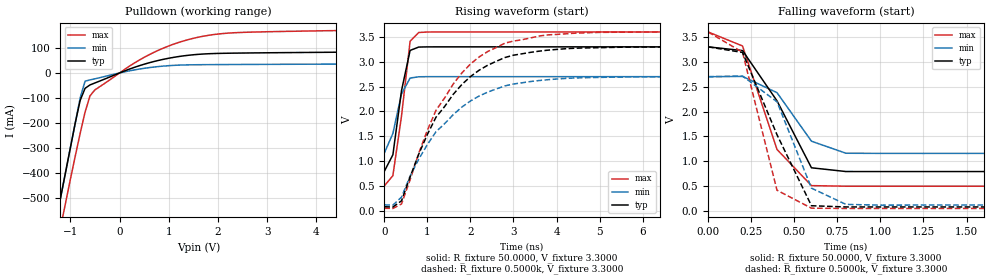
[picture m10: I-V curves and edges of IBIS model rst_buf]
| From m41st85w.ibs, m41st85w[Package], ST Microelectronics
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|   Model rst_buf
[Model]   rst_buf
Model_type   Open_drain
Polarity   Inverting
Vmeas =   1.5000V
Cref =  50.0000pF
Rref =   0.3330k
Vref =   1.7300V
C_comp   4.5300pF   4.4100pF   4.6100pF
[Temperature Range]   27.0000   85.0000   -40.0000
[Voltage Range]   3.2000V   2.7000V   3.6000V
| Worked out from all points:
|   slope of the pulldown table from 0 to 0.48 V, typ, clamps not added: 14.3 ohm
|   rising waveform, R_fixture 50.0000, V_fixture 3.3000: 20-80 % time 268ps typ, 270ps min, 274ps max; typ from 0.793 V to 3.3 V
|   rising waveform, R_fixture 0.5000k, V_fixture 3.3000: 20-80 % time 1.33ns typ, 1.39ns min, 1.28ns max; typ from 0.081 V to 3.3 V
|   falling waveform, R_fixture 50.0000, V_fixture 3.3000: 20-80 % time 252ps typ, 194ps min, 200ps max; typ from 3.3 V to 0.793 V
|   falling waveform, R_fixture 0.5000k, V_fixture 3.3000: 20-80 % time 249ps typ, 178ps min, 154ps max; typ from 3.3 V to 0.081 V
[Pulldown]
| voltage   I(typ)   I(min)   I(max)
-3.2V     -2.5A      -2.5A      -2.586A
-1.4V     -700mA     -700mA     -810.5mA
-1V       -300mA     -300mA     -425.7mA
-800mV    -109.6mA   -100mA     -241.4mA
-700mV    -61.27mA   -32.57mA   -156.4mA
-600mV    -47.64mA   -27.79mA   -91.21mA
-500mV    -39.89mA   -23.29mA   -67.59mA
100mV     7.894mA    4.371mA    13.86mA
800mV     50.46mA    25.78mA    91.43mA
1.5V      72.58mA    32.65mA    138.2mA
2.5V      79.48mA    33.9mA     161.8mA
6.4V      86.87mA    37.52mA    176.6mA
[Ramp]
| variable   typ   min   max
dV/dt_r   1.8493/0.8552n   1.5128/0.8949n   2.1145/0.8166n
dV/dt_f   1.8493/0.1573n   1.5128/0.1945n   2.1145/0.1081n
R_load = 0.3330k
[Rising Waveform]
R_fixture = 50.0000
V_fixture = 3.3000
V_fixture_min = 2.7000
V_fixture_max = 3.6000
| time   V(typ)   V(min)   V(max)
0s        793mV      1.158V     498.3mV
200ps     1.127V     1.557V     707.5mV
400ps     2.417V     2.352V     1.905V
600ps     3.228V     2.672V     3.412V
800ps     3.296V     2.698V     3.589V
1.2ns     3.3V       2.7V       3.6V
10ns      3.3V       2.7V       3.6V
[Rising Waveform]
R_fixture = 0.5000k
V_fixture = 3.3000
V_fixture_min = 2.7000
V_fixture_max = 3.6000
| time   V(typ)   V(min)   V(max)
0s        81.1mV     119mV      50.58mV
200ps     75.58mV    113.6mV    46.35mV
400ps     200.3mV    273.9mV    136.1mV
1ns       1.536V     1.333V     1.619V
1.2ns     1.882V     1.59V      2.021V
1.6ns     2.343V     1.934V     2.55V
2.2ns     2.828V     2.309V     3.095V
2.8ns     3.085V     2.514V     3.374V
4.8ns     3.28V      2.681V     3.588V
10ns      3.3V       2.7V       3.6V
[Falling Waveform]
R_fixture = 50.0000
V_fixture = 3.3000
V_fixture_min = 2.7000
V_fixture_max = 3.6000
| time   V(typ)   V(min)   V(max)
0s        3.3V       2.7V       3.6V
200ps     3.225V     2.706V     3.318V
400ps     2.214V     2.38V      1.238V
600ps     868.6mV    1.403V     509.7mV
800ps     793.4mV    1.161V     498.3mV
10ns      793mV      1.158V     498.3mV
[Falling Waveform]
R_fixture = 0.5000k
V_fixture = 3.3000
V_fixture_min = 2.7000
V_fixture_max = 3.6000
| time   V(typ)   V(min)   V(max)
0s        3.3V       2.7V       3.6V
200ps     3.188V     2.714V     3.192V
400ps     1.533V     2.196V     417mV
600ps     105.6mV    459.1mV    56.14mV
800ps     81.1mV     132.6mV    50.58mV
1ns       81.1mV     117mV      50.58mV
10ns      81.1mV     119mV      50.58mV
